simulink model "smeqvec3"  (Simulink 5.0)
settings: Solver=ode45  StartTime=0.0  StopTime=12  MaxStep=.05  RelTol=1e-4  AbsTol=1e-4
InitFcn:
  | smvecdef3
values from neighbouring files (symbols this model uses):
  Bm = 0.10    (= 0.1)    [IMabc2.m]    (also in imabcparam.m = 0.01; IMabcrun0.m = 0.01; IMabcrun1.m = 0.001; IMcur0.m = 1e-06)
  H = 0.60    (= 0.6)    [IMabc2.m]    (also in IMcur0.m = 0.3; imdef0vec.m = 0.3; imdef1vec.m = 0.3; imdef2vec.m = 0.3)
  n0 = 0.98    [imdef0vec.m]    (also in imdef1vec.m = 0.978; imdef2vec.m; imdefrotflux.m; imdefSIvec1.m = 0.95)
  Ra = .95    (= 0.95)    [altwdgs.m]    (also in Ccurverun.m = 0.018)
  V = [Vas 0 0].'    [Actac.m]    (also in acttrcalc1.m = str2num(get(h,'string')); im3d.m = eval(get(hVs,'String')); IMabc2.m = [vas vbs vcs 0 0 0]'; IMabcf0.m = [vas vbs vcs 0 0 0]')
  wo = 2*pi*freq0    [calc0.m]    (also in IMabc2.m = 376.991118431; imabcparam.m = 376.991118431; IMabcrun0.m = 376.991118431; IMabcrun1.m = 376.991118431)
undefined symbols (not defined in the file or in its folder): delta0, fa0, fk0, L_1, phif0, Rf, Rkd, Rkq, vf0
libraries: simulink x1

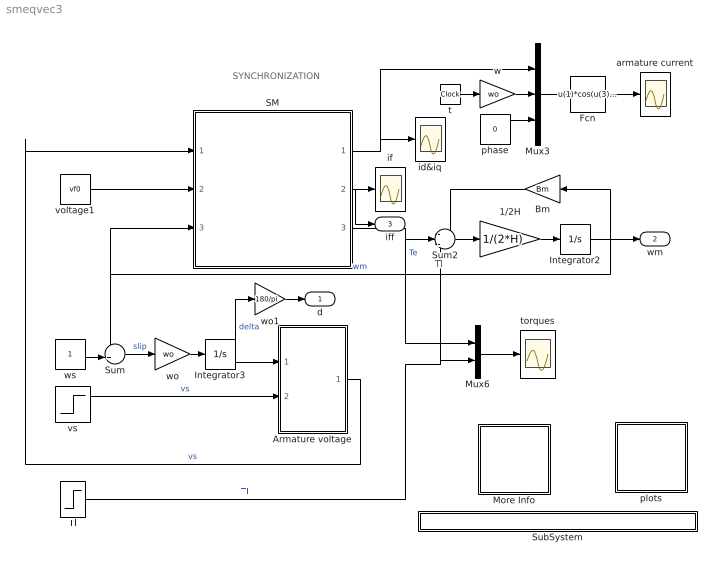
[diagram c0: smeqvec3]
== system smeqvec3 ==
  note: Tl
  note: SYNCHRONIZATION
  1/2H : Gain  Gain=1/(2*H)
  Armature voltage : Subsystem
  Bm : Gain  Orientation=left  Gain=Bm
  Fcn : Fcn  Expr=u(1)*cos(u(3)+u(4))+u(2)*sin(u(3)+u(4))
  Integrator2 : Integrator  InitialCondition=n0
  Integrator3 : Integrator  InitialCondition=delta0
  More Info : Subsystem
  Mux3 : Mux  Inputs=3
  Mux6 : Mux  Inputs=2
  SM : Subsystem
  SubSystem : Subsystem
  Sum : Sum  Inputs=-+|
  Sum2 : Sum  Inputs=-+-
  Tl : Step  Time=6  After=-1  SampleTime=0
  armature current : Scope
  id&iq : Scope
  if : Scope
  phase : Constant  Value=0
  plots : Subsystem
  t : Clock
  torques : Scope
  voltage1 : Constant  Value=vf0
  vs : Step  Time=0  After=V  SampleTime=0
  w : Gain  Gain=wo
  wo : Gain  Gain=wo
  wo1 : Gain  Gain=180/pi
  ws : Constant
  d : Outport
  wm : Outport  Port=2
  iff : Outport  Port=3
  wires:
  voltage1/1 -> SM/2(vf)
  1/2H/1 -> Integrator2/1
  Sum2/1 -> 1/2H/1
  Bm/1 -> Sum2/1
  SM/3(Te) -> Mux6/1, Sum2/2  "Te"
  Mux6/1 -> torques/1
  SM/1(ia) -> id&iq/1, Mux3/1
  SM/2(if) -> if/1, iff/1
  Integrator2/1 -> Bm/1, Sum/1, SM/3(wm), wm/1  "wm"
  w/1 -> Mux3/2
  phase/1 -> Mux3/3
  Mux3/1 -> Fcn/1
  t/1 -> w/1
  Fcn/1 -> armature current/1
  ws/1 -> Sum/2
  Sum/1 -> wo/1  "slip"
  Armature voltage/1(vs) -> SM/1(vs)  "vs"
  wo/1 -> Integrator3/1
  vs/1 -> Armature voltage/2(Vt)  "vs"
  Integrator3/1 -> Armature voltage/1(delta), wo1/1  "delta"
  wo1/1 -> d/1
  Tl/1 -> Mux6/2, Sum2/3  "Tl"

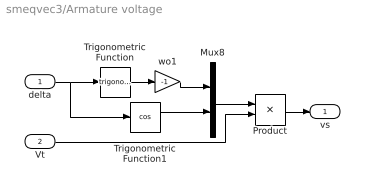
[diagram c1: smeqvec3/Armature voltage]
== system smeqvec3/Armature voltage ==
  delta : Inport
  Vt : Inport  Port=2
  Mux8 : Mux  Inputs=2
  Product : Product
  Trigonometric Function : Trigonometry
  Trigonometric Function1 : Trigonometry  Operator=cos
  wo1 : Gain  Gain=-1
  vs : Outport
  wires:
  delta/1 -> Trigonometric Function/1, Trigonometric Function1/1
  Trigonometric Function/1 -> wo1/1
  Mux8/1 -> Product/1
  wo1/1 -> Mux8/1
  Trigonometric Function1/1 -> Mux8/2
  Product/1 -> vs/1
  Vt/1 -> Product/2

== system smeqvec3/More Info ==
  note: ALTERNATOR SYNCHRONIZATION PROCESS

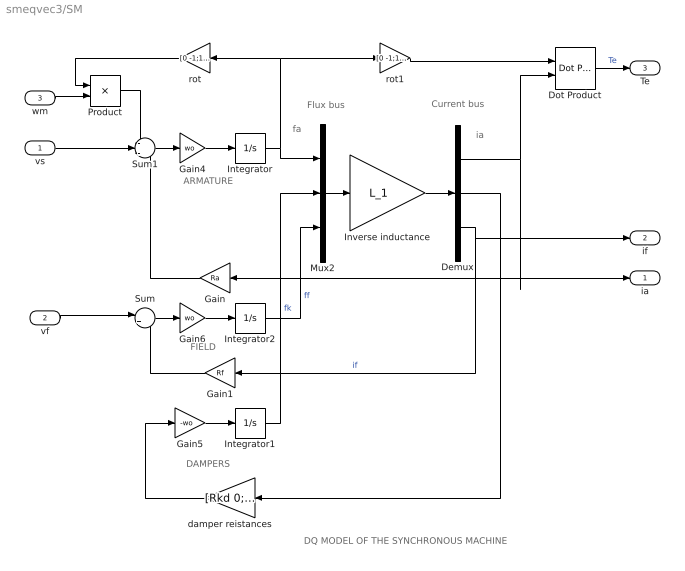
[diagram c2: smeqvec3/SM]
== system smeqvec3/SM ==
  note: DAMPERS
  note: ARMATURE
  note: fa
  note: ia
  note: FIELD
  note: DQ MODEL OF THE SYNCHRONOUS MACHINE
  note: Flux bus
  note: Current bus
  vs : Inport
  vf : Inport  Port=2
  wm : Inport  Port=3
  Demux : Demux  Outputs=3
  Dot Product : simulink/Math Operations/Dot Product
  Gain : Gain  Orientation=left  Gain=Ra
  Gain1 : Gain  Orientation=left  Gain=Rf
  Gain4 : Gain  Gain=wo
  Gain5 : Gain  Gain=-wo
  Gain6 : Gain  Gain=wo
  Integrator : Integrator  InitialCondition=fa0
  Integrator1 : Integrator  InitialCondition=fk0
  Integrator2 : Integrator  InitialCondition=phif0
  Inverse inductance : Gain  Gain=L_1  Multiplication=Matrix(K*u)
  Mux2 : Mux  Inputs=3
  Product : Product
  Sum : Sum  Inputs=|+-
  Sum1 : Sum  Inputs=-+-
  damper reistances : Gain  Orientation=left  Gain=[Rkd 0;0 Rkq]  Multiplication=Matrix(K*u)
  rot : Gain  Orientation=left  Gain=[0 -1;1 0]  Multiplication=Matrix(K*u)
  rot1 : Gain  Gain=[0 -1;1 0]  Multiplication=Matrix(K*u)
  ia : Outport
  if : Outport  Port=2
  Te : Outport  Port=3
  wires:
  Product/1 -> Sum1/1
  rot/1 -> Product/1
  wm/1 -> Product/2
  Gain5/1 -> Integrator1/1
  damper reistances/1 -> Gain5/1
  Integrator/1 -> Mux2/1, rot/1, rot1/1
  Sum1/1 -> Gain4/1
  Gain4/1 -> Integrator/1
  vs/1 -> Sum1/2
  Gain/1 -> Sum1/3
  Gain6/1 -> Integrator2/1
  Sum/1 -> Gain6/1
  vf/1 -> Sum/1
  Gain1/1 -> Sum/2
  rot1/1 -> Dot Product/1
  Demux/1 -> Gain/1, ia/1, Dot Product/2
  Dot Product/1 -> Te/1  "Te"
  Mux2/1 -> Inverse inductance/1
  Inverse inductance/1 -> Demux/1
  Integrator1/1 -> Mux2/2  "fk"
  Integrator2/1 -> Mux2/3  "ff"
  Demux/2 -> damper reistances/1
  Demux/3 -> if/1, Gain1/1  "if"

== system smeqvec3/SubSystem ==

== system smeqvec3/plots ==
